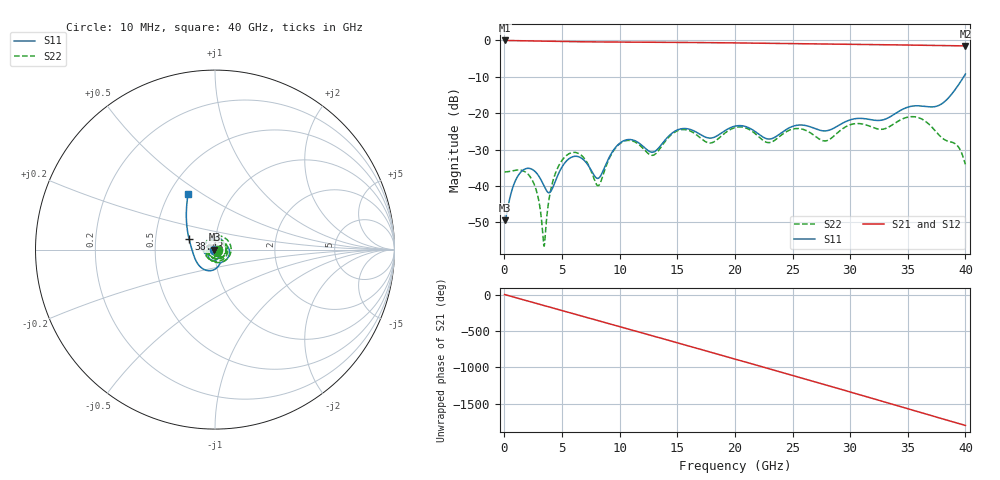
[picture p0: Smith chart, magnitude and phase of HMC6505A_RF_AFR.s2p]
! Analog Devices, Inc.
! 1 Analog Way
! Wilmington, MA 01887
! http://www.analog.com
! Date:  2021-09-17 NN
! Board Name:  EV1HMC6505ALC5 (125487-1) with HMC6505ALC5 installed
! File Description:  Automatic Fixture Removal S-Parameters for RF Port connector and board loss de-embedding
! File Generation:  Calibrated Network Analyzer
! Chip Part Number:  HMC6505A
! Chip Description:  GaAs, MMIC, IQ Upconverter
! Chip Frequency:  5.5 to 8.6 GHz
! Chip Package:  LCC, 4.9 x 4.9 x 1 mm
! RF Port:  HMC6505ALC5 removed and end of trace left open
! Note:
!  Analog Devices supplies this data as a sample of measured data at the evaluation board
!  ports for this product.  Your particular data for this product may vary.
!  Analog Devices reserves the right to change this data at anytime.
!  All lines below in this file are as is from the Network Analyzer.
!Agilent Technologies,N5245A,MY52451809,A.10.47.06
!Automatic Fixture Removal (AFR)
!Date: Friday, September 17, 2021 3:12:07 AM
!S2P File: Measurements: S11,S21,S12,S22:
# MHz S  RI  R 50
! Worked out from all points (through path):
!   4000 points, 10 MHz to 40 GHz, reference 50 ohm
!   highest |S21| = 0.00 dB at 10 MHz (marker M1); lowest = -1.5 dB at 40 GHz (marker M2)
!   group delay of S21, straight-line fit = 125 ps
!   lowest |S11| = -49.4 dB at 10 MHz (marker M3), VSWR 1.01, Z = 49.7 + j0.0162 ohm
!   |S11| at or under -10 dB: start of sweep to 39.85 GHz
!   |S22| runs from -56.5 to -20.9 dB; largest |S21 - S12| = 1.5e-15
!   S11 on the Smith chart (normalised r, x): 10 MHz: 0.99, +0.00; 38.43 GHz: 0.74, +0.09; 40 GHz: 0.62, +0.44
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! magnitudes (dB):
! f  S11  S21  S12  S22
! 10 MHz  -49.4  0.0  0.0  -36.1
! 1.06 GHz  -37.8  -0.1  -0.1  -35.6
! 2.3 GHz  -35.3  -0.1  -0.1  -37.8
! 2.88 GHz  -36.8  -0.2  -0.2  -42.6
! 3.43 GHz  -40.0  -0.2  -0.2  -56.5
! 4.01 GHz  -41.5  -0.2  -0.2  -41.1
! 4.63 GHz  -37.0  -0.3  -0.3  -34.9
! 5.62 GHz  -32.4  -0.3  -0.3  -31.1
! 6.68 GHz  -32.3  -0.4  -0.4  -31.6
! 8.12 GHz  -37.9  -0.4  -0.4  -39.9
! 10.21 GHz  -27.8  -0.4  -0.4  -27.9
! 13.34 GHz  -29.7  -0.5  -0.5  -30.3
! 15.15 GHz  -24.4  -0.5  -0.5  -24.6
! 17.85 GHz  -26.8  -0.6  -0.6  -28.2
! 20.01 GHz  -23.5  -0.7  -0.7  -23.9
! 22.95 GHz  -27.1  -0.8  -0.8  -28.1
! 25.08 GHz  -23.5  -0.8  -0.8  -24.3
! 26.67 GHz  -23.9  -0.9  -0.9  -25.6
! 33.34 GHz  -21.2  -1.2  -1.2  -23.8
! 35.78 GHz  -17.9  -1.3  -1.3  -21.1
! 38.43 GHz  -16.1  -1.4  -1.4  -27.6
! 40 GHz  -9.2  -1.5  -1.5  -34.0
